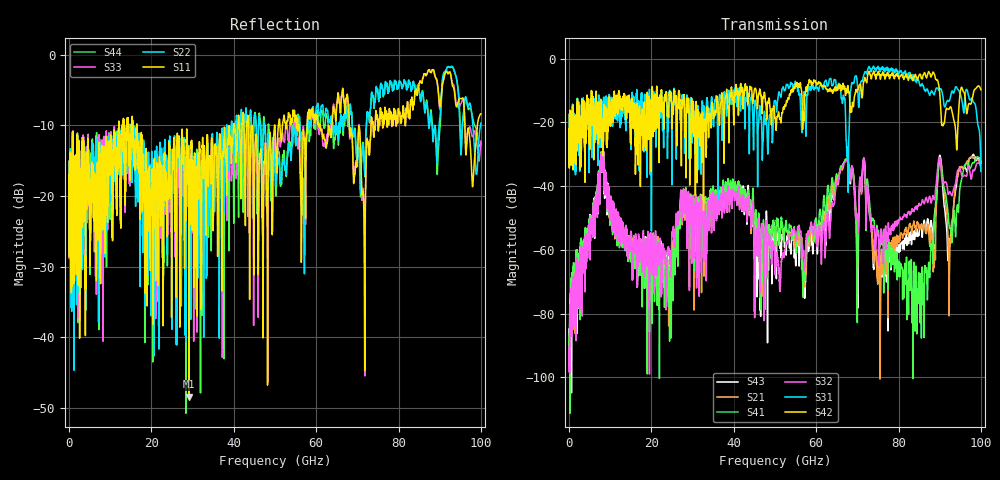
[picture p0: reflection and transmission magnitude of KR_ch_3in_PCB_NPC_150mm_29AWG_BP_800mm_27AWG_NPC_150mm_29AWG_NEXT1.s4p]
# GHz S RI R 45
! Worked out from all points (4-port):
!   4000 points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, 25 MHz to 100 GHz, reference 45 ohm
!   strongest paths, dB at 25 MHz, 25.02 GHz, 50.02 GHz, 75.03 GHz, 100 GHz:
!     S42: -22.2, -20.8, -18.7, -4.1, -9.8
!     S31: -22.1, -21.8, -13.4, -2.4, -35.4
!     S32: -89.9, -55.8, -67.7, -55.3, -34.2
!     S41: -88.5, -65.6, -58.6, -54.4, -31.9
!     S21: -89.7, -60.5, -58.1, -68.7, -32.8
!     S43: -91.7, -59.5, -59.5, -68.0, -32.3
!   lowest |S11| = -48.4 dB at 29.18 GHz (marker M1), VSWR 1.01, Z = 44.8 + j0.258 ohm
!   |S11| at or under -10 dB: start of sweep to 12.08 GHz; 16.48 GHz to 39.96 GHz (23.48 GHz wide, 83.2 % of centre); 44.45 GHz to 49.91 GHz (5.458 GHz wide, 11.6 % of centre)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
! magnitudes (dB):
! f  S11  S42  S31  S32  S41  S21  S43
! 25 MHz  -17.4  -22.2  -22.1  -89.9  -88.5  -89.7  -91.7
! 8.025 GHz  -15.7  -27.9  -17.6  -31.3  -31.1  -31.6  -30.9
! 29.18 GHz  -48.4  -16.4  -31.4  -55.5  -48.7  -52.2  -50.3
! 57.12 GHz  -11.9  -13.5  -10.8  -66.4  -68.9  -70.5  -69.0
! 67.33 GHz  -6.2  -9.6  -25.6  -31.9  -31.5  -31.7  -31.6
! 84.8 GHz  -5.0  -5.8  -6.7  -46.2  -70.1  -51.6  -54.9
! 100 GHz  -8.4  -9.8  -35.4  -34.2  -31.9  -32.8  -32.3
